ORGANIZATION_BLOCK MAIN:OB1
TITLE=

BEGIN
NETWORK 1
LD SM0.1
R M0.0 2

NETWORK 2
LDN C0
AN M0.0
A I0.1
A I0.0
O Q0.0
AN I0.6
A I0.7
A I0.3
= Q0.0

NETWORK 3
LD I0.4
S M0.0 1

NETWORK 4
LDN I0.2
R M0.0 1

NETWORK 5
LD I0.0
A M0.0
O I0.4
O Q0.1
A I0.2
A I0.7
AN I0.5
= Q0.1

NETWORK 6
LD I0.4
LD I1.4
LD SM0.1
CTUD C0 +6

NETWORK 7
LD I1.1
AN M0.1
A I1.0
O Q0.7
AN I1.5
A I1.7
A I1.3
= Q0.7

NETWORK 8
LD I1.4
ED
S M0.1 1

NETWORK 9
LDN I1.2
R M0.1 1

NETWORK 10
LD I1.4
ED
LD I1.0
A M0.1
OLD
O Q0.6
AN I1.6
A I1.7
A I1.2
= Q0.6

NETWORK 11
LD I0.2
A SM0.5
= Q1.0

NETWORK 12
LD I1.2
A SM0.5
= Q1.1

NETWORK 13
LD C0
= Q0.3

NETWORK 14
LDN C0
= Q0.2

NETWORK 15
LDN I1.3
= Q0.4

NETWORK 16
LD I1.3
= Q0.5

END_ORGANIZATION_BLOCK

